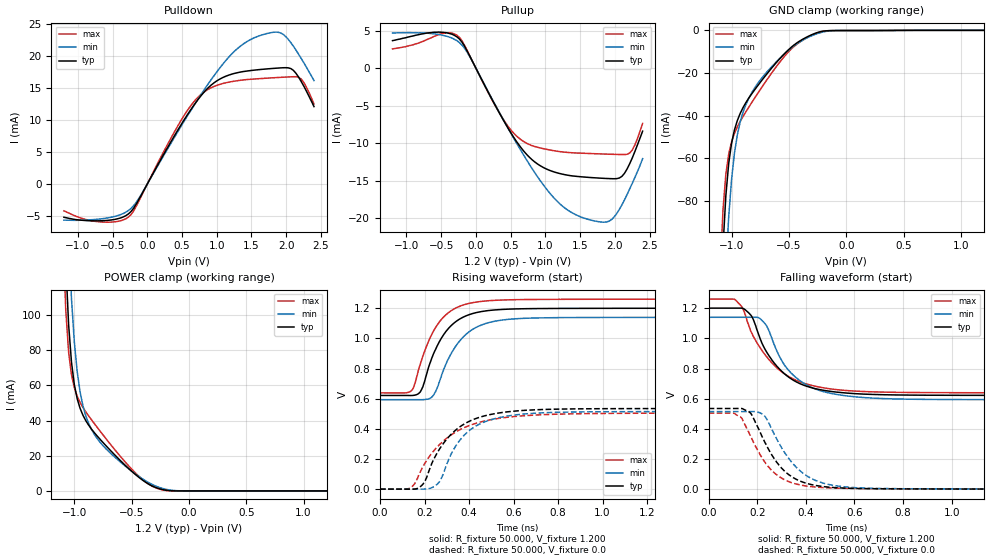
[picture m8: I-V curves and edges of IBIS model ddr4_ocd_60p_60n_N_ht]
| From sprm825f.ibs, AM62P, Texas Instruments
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|   Model ddr4_ocd_60p_60n_N_ht
[Model] ddr4_ocd_60p_60n_N_ht
Model_type I/O
Polarity   Non-Inverting
Enable   Active-High
Vinl =  0.700V
Vinh =  0.900V
Vmeas =  0.600V
C_comp   3.071pF   3.048pF   3.116pF
C_comp_pullup   0.296pF   0.292pF   0.302pF
C_comp_pulldown   1.212pF   1.204pF   1.227pF
[Model Spec]
Vinh   0.900V   0.820V   0.980V
Vinl   0.700V   0.620V   0.780V
Vmeas   0.600V   NA   NA
[Temperature Range]   25.000   0.125k   -40.000
[Voltage Range]   1.200V   1.140V   1.260V
[Pullup Reference]   1.200V   1.140V   1.260V
[Pulldown Reference]   0.0V   0.0V   0.0V
[C Comp Corner]
C_comp_pullup   0.292pF   0.296pF   0.302pF
C_comp_pulldown   1.204pF   1.212pF   1.227pF
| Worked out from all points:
|   slope of the pulldown table from 0 to 0.18 V, typ, clamps not added: 50.6 ohm
|   slope of the pullup table from 0 to 0.18 V, typ, clamps not added: 55.4 ohm
|   GND clamp passes 1 mA (typ) near -0.25 V on its own axis
|   POWER clamp passes 1 mA (typ) near -0.24 V on its own axis
|   rising waveform, R_fixture 50.000, V_fixture 1.200: 20-80 % time 115ps typ, 125ps min, 114ps max; typ from 0.622 V to 1.2 V
|   rising waveform, R_fixture 50.000, V_fixture 0.0: 20-80 % time 158ps typ, 139ps min, 196ps max; typ from 0.002 V to 0.536 V
|   falling waveform, R_fixture 50.000, V_fixture 1.200: 20-80 % time 141ps typ, 138ps min, 159ps max; typ from 1.2 V to 0.622 V
|   falling waveform, R_fixture 50.000, V_fixture 0.0: 20-80 % time 124ps typ, 135ps min, 118ps max; typ from 0.536 V to 0.002 V
[Pulldown]
|Voltage   I(typ)   I(min)   I(max)
-1.2V     -5.186mA   -5.633mA   -4.184mA
-643mV    -5.726mA   -5.406mA   -5.937mA
-235mV    -4.303mA   -3.816mA   -4.781mA
396mV     7.636mA    7.389mA    8.249mA
693mV     12.66mA    12.63mA    13.14mA
1.027V    16.29mA    17.9mA     15.52mA
1.472V    17.71mA    22.49mA    16.36mA
1.806V    18.06mA    23.7mA     16.6mA
1.955V    18.17mA    23.4mA     16.69mA
2.103V    17.77mA    21.54mA    16.77mA
2.214V    16.06mA    19.65mA    16.43mA
2.4V      12.1mA     16.17mA    12.5mA
[Pullup]
|Voltage   I(typ)   I(min)   I(max)
-1.2V     3.673mA    4.689mA    2.574mA
-532mV    4.814mA    4.494mA    4.499mA
-235mV    3.869mA    3.401mA    4.084mA
322mV     -5.7mA     -5.628mA   -5.713mA
581mV     -9.73mA    -9.937mA   -9.014mA
915mV     -12.95mA   -14.85mA   -10.61mA
1.175V    -13.97mA   -17.8mA    -11.08mA
1.435V    -14.42mA   -19.53mA   -11.31mA
1.955V    -14.74mA   -20.17mA   -11.48mA
2.103V    -14.42mA   -18.21mA   -11.52mA
2.214V    -12.74mA   -16.1mA    -11.32mA
2.4V      -8.403mA   -12.07mA   -7.368mA
[GND_clamp]
|Voltage   I(typ)   I(min)   I(max)
-1.2V     -425.9mA   -479.1mA   -398.3mA
-1.1V     -138.2mA   -191.6mA   -113.7mA
-1.075V   -101.6mA   -146.5mA   -84.28mA
-1.05V    -77.49mA   -112.3mA   -67.47mA
-1.025V   -62.34mA   -87.34mA   -58.02mA
-1V       -52.87mA   -69.78mA   -52.27mA
-975mV    -46.68mA   -57.59mA   -48.3mA
-900mV    -36.21mA   -38.39mA   -40.36mA
-750mV    -24.4mA    -23.28mA   -27.78mA
-425mV    -5.686mA   -6.132mA   -6.273mA
-175mV    -233uA     -499.3uA   -237.7uA
1.2V      0A         0A         0A
[POWER_clamp]
|Voltage   I(typ)   I(min)   I(max)
-1.2V     676.6mA    754.8mA    654.2mA
-1.1V     185.8mA    267.5mA    148mA
-1.075V   130.1mA    197.5mA    103.3mA
-1.05V    94.76mA    146mA      79.03mA
-1.025V   73.36mA    109.6mA    66.12mA
-1V       60.47mA    84.71mA    58.72mA
-975mV    52.41mA    67.84mA    53.9mA
-925mV    43.07mA    48.41mA    47.45mA
-775mV    29.35mA    27.65mA    33.98mA
-400mV    5.928mA    6.639mA    6.211mA
-125mV    43.28uA    213.5uA    14.43uA
1.2V      0A         0A         0A
[Ramp]
| variable   typ   min   max
dV/dt_r   0.381/0.163n   0.355/0.171n   0.406/0.196n
dV/dt_f   0.380/0.147n   0.355/0.156n   0.406/0.132n
R_load = 60.000
[Rising Waveform]
R_fixture= 50.000
V_fixture= 1.200
V_fixture_min= 1.140
V_fixture_max= 1.260
|time   V(typ)   V(min)   V(max)
0s        622mV      594.1mV    639.1mV
144ps     621.8mV    594.1mV    657.9mV
182ps     648.4mV    593.8mV    834.7mV
229ps     853.8mV    606.7mV    1.016V
276ps     1.002V     751.8mV    1.126V
317ps     1.08V      892.4mV    1.18V
368ps     1.136V     1V         1.218V
437ps     1.172V     1.076V     1.241V
687ps     1.197V     1.134V     1.257V
3ns       1.2V       1.14V      1.26V
[Rising Waveform]
R_fixture= 50.000
V_fixture= 0.0
V_fixture_min= 0.0
V_fixture_max= 0.0
|time   V(typ)   V(min)   V(max)
0s        2.043mV    2.432mV    3.486mV
129ps     1.971mV    2.399mV    5.877mV
174ps     11.45mV    2.356mV    94.27mV
202ps     54.8mV     2.615mV    174.3mV
246ps     212.8mV    21.98mV    263.3mV
278ps     291mV      81.03mV    312mV
309ps     348.5mV    200mV      349.7mV
388ps     441.2mV    373.1mV    415.3mV
568ps     512.9mV    484.7mV    477mV
3ns       536mV      515.9mV    505.7mV
[Falling Waveform]
R_fixture= 50.000
V_fixture= 1.200
V_fixture_min= 1.140
V_fixture_max= 1.260
|time   V(typ)   V(min)   V(max)
0s        1.2V       1.139V     1.26V
114ps     1.2V       1.139V     1.248V
138ps     1.199V     1.139V     1.205V
174ps     1.153V     1.139V     1.045V
208ps     1.015V     1.134V     947mV
260ps     856.8mV    1.001V     838.3mV
339ps     732.9mV    771mV      738.6mV
500ps     649.5mV    636.9mV    665.9mV
900ps     623.7mV    596mV      641mV
3ns       622mV      593.8mV    639.1mV
[Falling Waveform]
R_fixture= 50.000
V_fixture= 0.0
V_fixture_min= 0.0
V_fixture_max= 0.0
|time   V(typ)   V(min)   V(max)
0s        535.8mV    515.2mV    505.4mV
130ps     536.2mV    515.3mV    481.3mV
174ps     502.5mV    515.3mV    347.3mV
221ps     346.1mV    498.8mV    206.4mV
269ps     205.2mV    368.6mV    112.1mV
329ps     98.77mV    206.8mV    52.45mV
399ps     42.49mV    95.08mV    23.6mV
479ps     17.85mV    38.87mV    11.71mV
809ps     3.705mV    4.399mV    4.742mV
3ns       2.022mV    2.258mV    3.477mV
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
